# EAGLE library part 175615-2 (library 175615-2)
TE Connectivity Mark II Series 16 Way 2 Row Female Right Angle PCB Housing Source: Datasheet
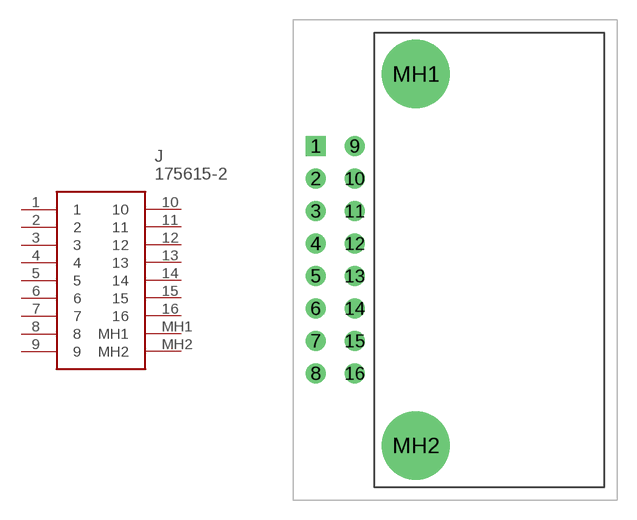
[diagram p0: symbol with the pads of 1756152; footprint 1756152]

Designator prefix J

## 175615-2 (Description: TE Connectivity Mark II Series 16 Way 2 Row Female Right Angle PCB Housing; Height: 16.9mm; Manufacturer_Name: TE Connectivity; Manufacturer_Part_Number: 175615-2; Mouser_Part_Number: 571-175615-2; Mouser_Price-Stock: https://www.mouser.co.uk/ProductDetail/TE-Connectivity-AMP/175615-2/?qs=Boq%252BepwQt6qz7faZSh%252BOMQ%3D%3D)  [1756152]
1  1
2  2
3  3
4  4
5  5
6  6
7  7
8  8
9  9
10  10
11  11
12  12
13  13
14  14
15  15
16  16
MH1  MH1
MH2  MH2

## Footprint 1756152 (pad centres in mm)
175615-2-3
drill 1 pad 1.5 square: 1 -3,0
drill 1 pad 1.5: 2 -3,-2.5; 3 -3,-5; 4 -3,-7.5; 5 -3,-10; 6 -3,-12.5; 7 -3,-15; 8 -3,-17.5; 9 0,0; 10 0,-2.5; 11 0,-5; 12 0,-7.5; 13 0,-10; 14 0,-12.5; 15 0,-15; 16 0,-17.5
drill 3.5 pad 5.25: MH1 4.7,5.55; MH2 4.7,-23.05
